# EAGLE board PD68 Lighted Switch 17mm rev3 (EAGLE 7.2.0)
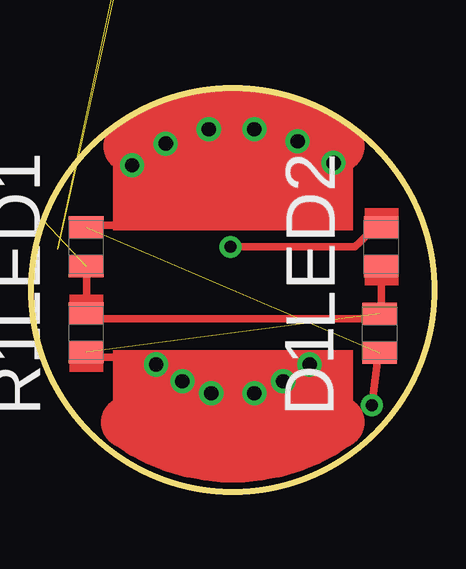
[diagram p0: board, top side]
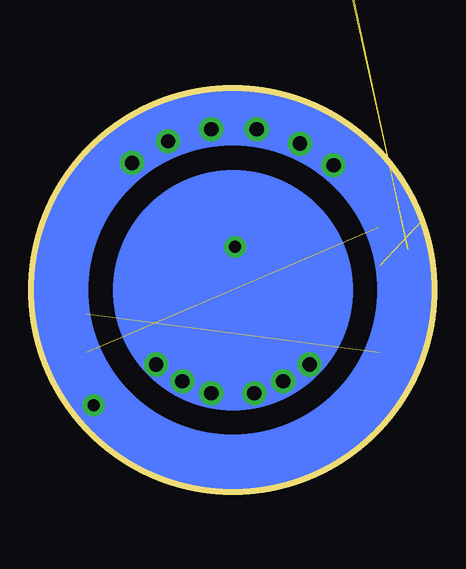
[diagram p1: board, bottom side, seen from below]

No outline drawn. Coordinates in mm, seen from the top.
Copper layers (1*16): Top 0.035mm / dielectric 1.5mm / Bottom 0.035mm
Design rules "default *": minimum track width 10mil, minimum drill 24mil, track to track 8mil, track to pad 8mil, pad to pad 8mil, via to via 8mil, smd to smd 8mil, copper to edge 40mil, drill to drill 8mil, minimum pad ring 10mil, minimum via ring 8mil, stop-mask expansion 4mil, vias tented up to drill 60mil, thermal gap 10mil
Milling: area 14.5,0.7 to 31.3,17.5; area 14.5,0.7 to 31.3,17.5

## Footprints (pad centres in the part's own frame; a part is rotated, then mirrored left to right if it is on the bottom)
CAPC2013X94N = smd 0.914 x 1.448: 1 -0.813,0; 2 0.813,0

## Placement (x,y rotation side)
D1  10pF  [CAPC2013X94N]  29.02,7.3 90 top
LED1  10pF  [CAPC2013X94N]  16.78,10.9 90 top
LED2  10pF  [CAPC2013X94N]  29.08,10.9 90 top
R1  10pF  [CAPC2013X94N]  16.78,7.32 90 top

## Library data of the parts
D1 LED1 LED2 R1 = C_0805; MPN: 08051A100JAT2A; OC_FARNELL: 499158; OC_NEWARK: 96K4767; SUPPLIER: AVX; TOLERANCE: ±5%; VOLTAGERATING: 100V

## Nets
BATT+: LED1.1
BATT-: R1.2
N$1: D1.1 LED1.2
N$2: D1.2 R1.1

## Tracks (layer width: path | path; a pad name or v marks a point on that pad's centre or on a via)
BATT+  (1 unrouted)
N$1  (1 unrouted)
N$2  (1 unrouted)
S$1
  Top 0.305: 18.2,11.8 16.8,11.8
S$3  (6 unrouted)
S$5
  Top 0.305: 16.8,6.3 18.6,6.3
S$6  (via drill 0.6)
  other vias: 18.7,14.3
S$7
  Top 0.305: 16.8,8.2 16.8,7.9 29,7.9 | 16.8,8.2 16.8,10.3 | 16.8,8.2 16.9,8.2
S$8  (via drill 0.6)
  Top 0.305: v27.1,14.4 27.1,12.4
S$9
  Top 2.184: 18.5,3.6 arc72 27.3,3.6 | 27.3,15.1 arc72 18.6,15.1
S$10
  Top 0.305: 29.1,9.6 29.1,8
S$11  (via drill 0.5)
  Top 0.305: v28.7,4.3 29,6.6
S$12  (via drill 0.6)
  other vias: 20.1,15.2
S$13  (via drill 0.6)
  other vias: 21.9,15.8
S$14  (via drill 0.6)
  other vias: 23.8,15.8
S$15  (via drill 0.6)
  other vias: 25.6,15.3
S$16  (via drill 0.6)
  other vias: 26.1,6
S$17  (via drill 0.6)
  other vias: 19.7,6
S$18  (via drill 0.6)
  other vias: 25,5.3
S$19  (via drill 0.6)
  other vias: 20.8,5.3
S$20  (via drill 0.6)
  other vias: 22,4.8
S$21  (via drill 0.6)
  other vias: 23.8,4.8
S$22  (via drill 0.5)
  Top 0.305: 28.9,11.8 28.2,11.1 28,10.9 v22.8,10.9
(copper drawn outside any net)
  shapes: Bottom circle x2, Top area x6

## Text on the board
tTest(labels): + | LED | R | R | BLF | LED | +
